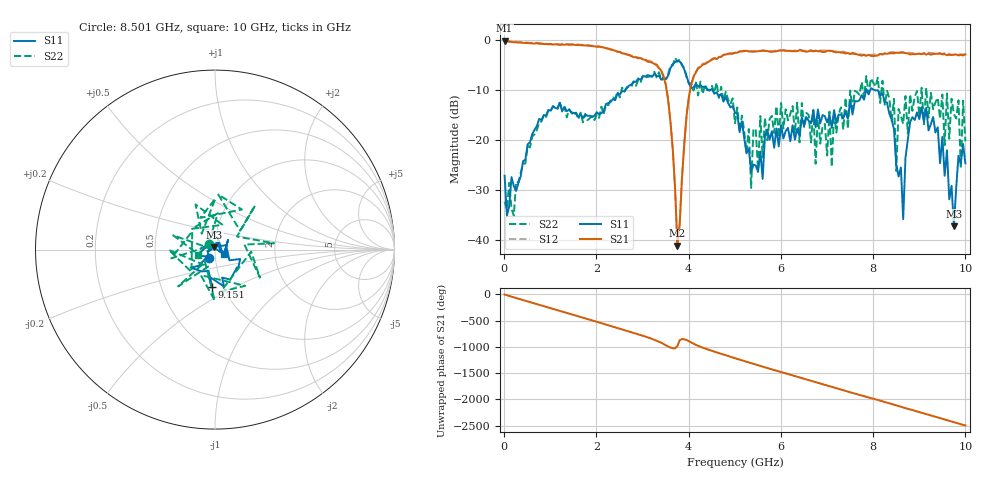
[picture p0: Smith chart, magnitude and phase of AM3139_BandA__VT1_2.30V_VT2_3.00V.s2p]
! Date/Time: Tue, Nov 13, 2018 4:57 PM
! Network Analyzer: Agilent Technologies E8364B Rev: A.07.50.67
! Sweep from 0.010 to 10.000 GHz, 201 Points, Sweep Type: LIN
! Power Supply: 2.301 V, 0.000 A
# Hz S DB R 50
!freq MagS11 AngS11 MagS21 AngS21 MagS12 AngS12 MagS22 AngS22
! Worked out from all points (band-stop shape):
!   201 points, 10 MHz to 10 GHz, reference 50 ohm
!   highest |S21| = -0.16 dB at 10 MHz (marker M1); lowest = -41.2 dB at 3.756 GHz (marker M2)
!   |S21| within 3 dB of the highest: start of sweep to 2.729 GHz; 4.738 GHz to 7.745 GHz (3.008 GHz wide, 48.2 % of centre)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
!   lowest |S11| = -37.4 dB at 9.75 GHz (marker M3), VSWR 1.03, Z = 49.5 + j1.27 ohm
!   |S11| at or under -10 dB: start of sweep to 2.635 GHz; 4.515 GHz to 7.848 GHz (3.333 GHz wide, 53.9 % of centre); 8.018 GHz to end of sweep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
!   |S22| runs from -35.2 to -3.6 dB; largest |S21 - S12| = 0.034
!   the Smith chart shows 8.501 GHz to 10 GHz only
!   S11 on the Smith chart (normalised r, x): 8.501 GHz: 0.93, -0.09; 9.151 GHz: 0.89, -0.39; 10 GHz: 1.11, -0.06
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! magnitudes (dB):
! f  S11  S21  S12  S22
! 10 MHz  -27.2  -0.2  -0.1  -32.4
! 1.708 GHz  -15.7  -1.1  -1.1  -16.5
! 3.357 GHz  -7.2  -5.7  -5.7  -6.5
! 3.606 GHz  -5.7  -16.5  -16.4  -5.1
! 3.756 GHz  -4.2  -41.2  -41.3  -4.4
! 4.106 GHz  -9.5  -7.4  -7.5  -10.2
! 5.005 GHz  -14.6  -2.6  -2.5  -16.7
! 5.305 GHz  -21.8  -2.3  -2.3  -17.9
! 5.355 GHz  -26.4  -2.4  -2.2  -29.7
! 5.554 GHz  -22.3  -2.3  -2.2  -15.3
! 6.703 GHz  -14.2  -2.3  -2.3  -14.0
! 6.753 GHz  -17.5  -2.2  -2.3  -24.8
! 7.053 GHz  -15.1  -2.2  -2.2  -14.4
! 7.103 GHz  -17.6  -2.2  -2.3  -25.4
! 7.502 GHz  -12.1  -2.9  -2.8  -10.2
! 8.352 GHz  -14.8  -2.7  -2.6  -11.8
! 8.501 GHz  -25.0  -2.6  -2.4  -26.3
! 8.651 GHz  -35.9  -2.5  -2.6  -16.8
! 8.801 GHz  -16.5  -2.9  -2.6  -10.9
! 9.151 GHz  -13.6  -3.0  -2.8  -9.6
! 9.75 GHz  -37.4  -3.0  -3.0  -14.9
! 10 GHz  -24.7  -2.9  -2.8  -20.3
